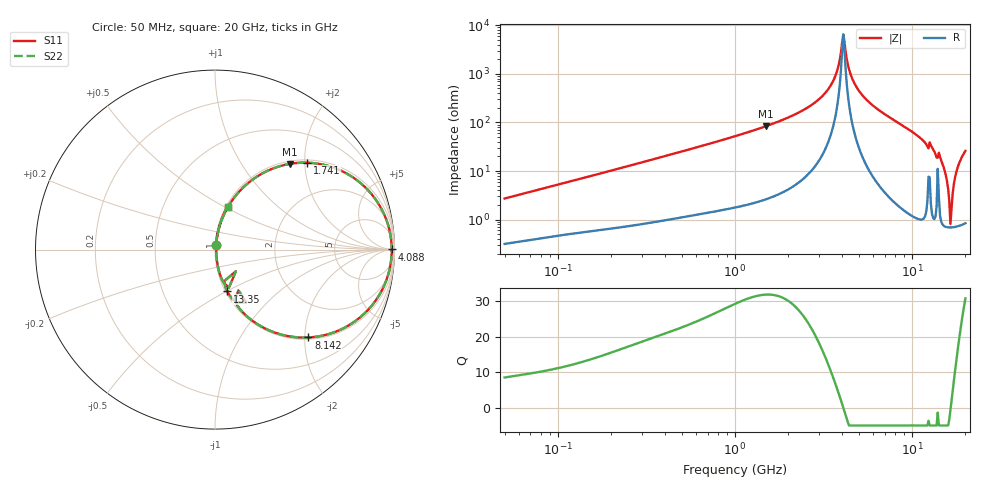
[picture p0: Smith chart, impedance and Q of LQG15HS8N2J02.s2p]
!Murata Part Number: LQG15HS8N2J02
!These Parameters are Measured in Series Mode Connection
!  o--[Z]--o
!Port1  Port2
!  o-------o
!Freq. Start=50[MHz] Stop=20[GHz], 401[Steps]
# Hz S RI R 50
!Freq.(Hz) S11(Real) S11(Imag) S21(Real) S21(Imag) S12(Real) S12(Imag) S22(Real) S22(Imag)
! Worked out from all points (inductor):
!   401 points, 50 MHz to 20 GHz, reference 50 ohm
!   read as one part in series: L = 8.5 nH near 51.52 MHz
!   highest Q = 31.9 at 1.498 GHz (marker M1), where L = 8.92 nH
!   self-resonance near 4.088 GHz
!   S11 on the Smith chart (normalised r, x): 50 MHz: 1.01, +0.05; 1.741 GHz: 1.07, +2.05; 4.088 GHz: open; 8.142 GHz: 1.04, -2.09; 13.35 GHz: 1.02, -0.51; 20 GHz: 1.02, +0.52
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5e7  0.00388 0.0269  0.9961 -0.0269  0.9961 -0.0269  0.00388 0.0269
1.364002e8  0.0103 0.0693  0.9897 -0.0693  0.9897 -0.0693  0.0103 0.0693
3.721004e8  0.0423 0.1782  0.9577 -0.1782  0.9577 -0.1782  0.0423 0.1782
1e9  0.2211 0.3983  0.7789 -0.3983  0.7789 -0.3983  0.2211 0.3983
1.498439e9  0.4163 0.4775  0.5837 -0.4775  0.5837 -0.4775  0.4163 0.4775
1.740566e9  0.5133 0.4842  0.4867 -0.4842  0.4867 -0.4842  0.5133 0.4842
2.728004e9  0.8341 0.35  0.1659 -0.35  0.1659 -0.35  0.8341 0.35
3.519108e9  0.9606 0.1493  0.0394 -0.1493  0.0394 -0.1493  0.9606 0.1493
3.736399e9  0.9757 0.0916  0.0243 -0.0916  0.0243 -0.0916  0.9757 0.0916
4.087748e9  0.9848 0.000791  0.0152 -0.000791  0.0152 -0.000791  0.9848 0.000791
4.472136e9  0.9764 -0.0921  0.0236 0.0921  0.0236 0.0921  0.9764 -0.0921
4.966507e9  0.9437 -0.198  0.0563 0.198  0.0563 0.198  0.9437 -0.198
7.442007e9  0.619 -0.4746  0.381 0.4746  0.381 0.4746  0.619 -0.4746
8.141811e9  0.5207 -0.4897  0.4793 0.4897  0.4793 0.4897  0.5207 -0.4897
1.066139e10  0.2322 -0.4126  0.7678 0.4126  0.7678 0.4126  0.2322 -0.4126
1.334722e10  0.0684 -0.2329  0.9316 0.2329  0.9316 0.2329  0.0684 -0.2329
1.504638e10  0.0218 -0.1182  0.9782 0.1182  0.9782 0.1182  0.0218 -0.1182
1.646126e10  0.00689 -0.00428  0.9931 0.00428  0.9931 0.00428  0.00689 -0.00428
1.696185e10  0.00807 0.0337  0.9919 -0.0337  0.9919 -0.0337  0.00807 0.0337
1.747767e10  0.0123 0.0718  0.9877 -0.0718  0.9877 -0.0718  0.0123 0.0718
1.800918e10  0.0195 0.1098  0.9805 -0.1098  0.9805 -0.1098  0.0195 0.1098
2e10  0.0702 0.2397  0.9298 -0.2397  0.9298 -0.2397  0.0702 0.2397
